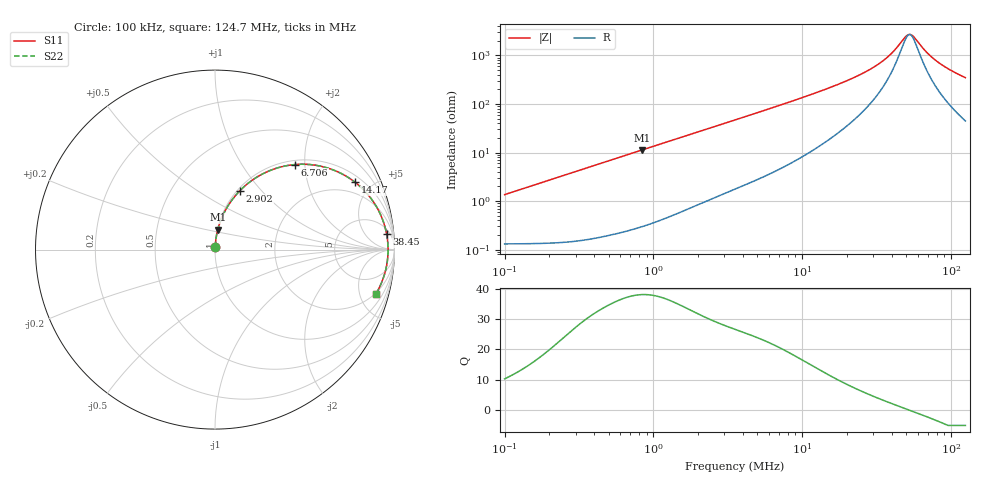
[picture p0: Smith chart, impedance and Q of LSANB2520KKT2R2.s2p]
! LSANB2520KKT2R2  S-PARAMETER MODEL  ( General Type )
! Model Generated by TAIYO YUDEN Corporation (http://www.ty-top.com)
! Version 2.0
! TAIYO YUDEN Control No. 20210629
! Copyright(c) 2013 TAIYO YUDEN CO.,LTD. All Rights Reserved.
! Product Description (link to TY-COMPAS)
! https://ds.yuden.co.jp/TYCOMPAS/or/detail?pn=LSANB2520KKT2R2M&u=M
! Products Name : Inductors
! Characteristics :
!  Inductance : 2.2 uH , SRF(min) : -Hz , DC Resistance(max) : 0.156 Ohm
!  Rated Current : Saturation :1900 mA , Temp Rise : 1500 mA (40 degC)
!  Case Size : 2.5 x 2.0 / 0.098 x 0.079 [mm/inch] , Thickness : 1 / 0.039 [mm/inch]
!  (Conditions: Temperature = 25 degC , DC Bias Current/Voltage = 0A / 0V)
! External Node Assignments :
!  1  o---GGG---o  2
! GND o---------o GND
! Frequency Range : 0.1MHz  -  124.6553MHz  [ 402 STEP ]
# MHz S RI R 50
! Freq[MHz].  S11 Real  S11 Imag  S21 Real  S21 Imag  S12 Real  S12 Imag  S22 Real  S22 Imag
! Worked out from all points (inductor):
!   401 points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, 100 kHz to 124.7 MHz, reference 50 ohm
!   read as one part in series: L = 2.15 uH near 103.6 kHz
!   highest Q = 38 at 833.6 kHz (marker M1), where L = 2.14 uH
!   self-resonance near 52.59 MHz
!   S11 on the Smith chart (normalised r, x): 100 kHz: 1.00, +0.03; 2.902 MHz: 1.03, +0.77; 6.706 MHz: 1.08, +1.78; 14.17 MHz: 1.32, +3.96; 38.45 MHz: 8, +19; 124.7 MHz: 1.89, -6.92
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0.1  0.00149 0.0135  0.9985 -0.0135  0.9985 -0.0135  0.00149 0.0135
0.330013  0.00352 0.0444  0.9965 -0.0444  0.9965 -0.0444  0.00352 0.0444
0.833631  0.0153 0.1102  0.9847 -0.1102  0.9847 -0.1102  0.0153 0.1102
1.089088  0.0246 0.1422  0.9754 -0.1422  0.9754 -0.1422  0.0246 0.1422
1.892259  0.0666 0.2342  0.9334 -0.2342  0.9334 -0.2342  0.0666 0.2342
2.902173  0.1383 0.3279  0.8617 -0.3279  0.8617 -0.3279  0.1383 0.3279
3.530656  0.189 0.3732  0.811 -0.3732  0.811 -0.3732  0.189 0.3732
6.706089  0.4459 0.4739  0.5541 -0.4739  0.5541 -0.4739  0.4459 0.4739
8.761097  0.5765 0.4673  0.4235 -0.4673  0.4235 -0.4673  0.5765 0.4673
11.65164  0.7056 0.4229  0.2944 -0.4229  0.2944 -0.4229  0.7056 0.4229
14.17487  0.7799 0.3757  0.2201 -0.3757  0.2201 -0.3757  0.7799 0.3757
19.53556  0.8703 0.2835  0.1297 -0.2835  0.1297 -0.2835  0.8703 0.2835
25.98091  0.9209 0.198  0.0791 -0.198  0.0791 -0.198  0.9209 0.198
32.17553  0.9444 0.1358  0.0556 -0.1358  0.0556 -0.1358  0.9444 0.1358
38.45196  0.9565 0.0856  0.0435 -0.0856  0.0435 -0.0856  0.9565 0.0856
49.34786  0.9641 0.0172  0.0359 -0.0172  0.0359 -0.0172  0.9641 0.0172
52.99385  0.9644 -0.00211  0.0356 0.00211  0.0356 0.00211  0.9644 -0.00211
55.90405  0.9641 -0.0166  0.0359 0.0166  0.0359 0.0166  0.9641 -0.0166
68.0104  0.9594 -0.0702  0.0406 0.0702  0.0406 0.0702  0.9594 -0.0702
79.84153  0.9506 -0.115  0.0494 0.115  0.0494 0.115  0.9506 -0.115
98.87811  0.931 -0.1767  0.069 0.1767  0.069 0.1767  0.931 -0.1767
124.6553  0.897 -0.2461  0.103 0.2461  0.103 0.2461  0.897 -0.2461
